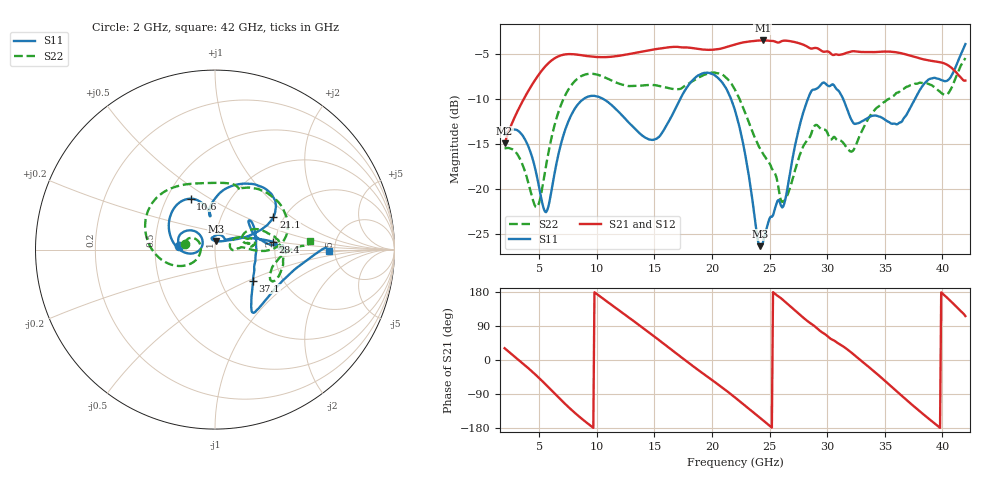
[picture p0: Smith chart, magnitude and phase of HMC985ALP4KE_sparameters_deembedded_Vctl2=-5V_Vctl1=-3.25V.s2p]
!s2p File: Measurements: S11, S21, S12, S22
# GHz S dB R 50.0
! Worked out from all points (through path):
!   401 points, 2 GHz to 42 GHz, reference 50 ohm
!   highest |S21| = -3.53 dB at 24.4 GHz (marker M1); lowest = -14.9 dB at 2 GHz (marker M2)
!   lowest |S11| = -26.3 dB at 24.2 GHz (marker M3), VSWR 1.10, Z = 50.6 + j4.82 ohm
!   |S11| at or under -10 dB: start of sweep to 8.878 GHz; 10.54 GHz to 17.26 GHz (6.714 GHz wide, 48.3 % of centre); 21.65 GHz to 28.33 GHz (6.681 GHz wide, 26.7 % of centre)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
!   |S22| runs from -22.0 to -5.5 dB; largest |S21 - S12| = 0.00065
!   S11 on the Smith chart (normalised r, x): 2 GHz: 0.67, +0.03; 10.6 GHz: 0.66, +0.41; 21.1 GHz: 1.76, +0.74; 28.4 GHz: 1.94, +0.19; 37.1 GHz: 1.42, -0.53; 42 GHz: 4.50, -0.10
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2  -13.97 173.8  -14.92 31.0  -14.93 31.0  -15.51 169.2
4.7  -18.00 135.7  -7.80 -39.2  -7.81 -39.2  -21.99 173.5
5.6  -22.57 164.8  -6.31 -65.6  -6.31 -65.6  -17.41 -150.1
7  -14.50 -178.0  -5.14 -108.4  -5.14 -108.4  -10.34 -169.5
8.7  -10.17 143.9  -5.17 -155.1  -5.17 -155.1  -7.45 155.0
10.6  -10.04 115.7  -5.38 160.7  -5.38 160.7  -7.57 124.9
13.2  -13.17 99.3  -4.94 102.9  -4.94 102.9  -8.58 90.0
15.4  -14.23 99.3  -4.44 52.6  -4.44 52.7  -8.56 70.9
18  -8.42 72.2  -4.32 -8.0  -4.32 -8.0  -8.30 63.7
21.1  -8.58 29.1  -4.32 -77.3  -4.32 -77.3  -7.51 15.8
22  -11.28 23.2  -3.97 -98.9  -3.97 -98.9  -9.00 3.5
24.2  -26.34 80.3  -3.53 -153.3  -3.53 -153.2  -15.57 3.4
24.4  -26.04 95.4  -3.52 -158.3  -3.53 -158.3  -16.03 4.4
26.2  -21.92 42.7  -3.55 157.5  -3.56 157.5  -21.39 14.1
28.4  -9.77 7.7  -4.31 100.2  -4.31 100.2  -14.40 18.3
28.7  -9.03 2.9  -4.42 94.1  -4.43 94.2  -13.55 17.4
30.6  -8.50 1.9  -5.13 51.3  -5.13 51.4  -14.21 10.5
32.4  -12.79 25.5  -4.73 11.9  -4.73 11.9  -15.42 26.1
35.4  -12.60 12.3  -4.76 -65.3  -4.77 -65.2  -9.97 15.7
37.1  -11.27 -39.1  -5.16 -111.0  -5.16 -111.0  -8.58 1.9
39.7  -7.80 -53.0  -5.90 -176.5  -5.91 -176.5  -9.13 -28.6
42  -3.93 -0.6  -7.97 115.9  -7.98 116.0  -5.47 4.9
